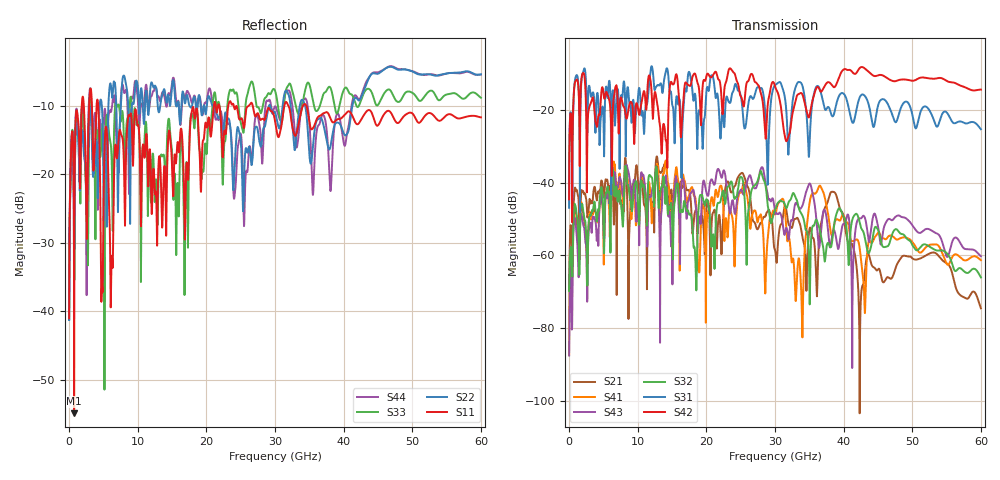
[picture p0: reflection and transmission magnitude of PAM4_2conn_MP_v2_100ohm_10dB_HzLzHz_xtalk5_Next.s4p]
! Info: Touchstone file created by Circ.  Input file=FAB50GbE_2conn_Midplane_Examax_Topo2_v2_100ohm_10dB_HzLzHz.circ
# Hz S RI R 50
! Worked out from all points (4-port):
!   6000 points, 10 MHz to 60 GHz, reference 50 ohm
!   strongest paths, dB at 10 MHz, 15.01 GHz, 30.01 GHz, 45.01 GHz, 60 GHz:
!     S42: -44.6, -12.9, -13.6, -10.6, -14.5
!     S31: -46.9, -18.4, -13.3, -19.0, -25.4
!     S32: -69.8, -50.1, -47.5, -53.0, -66.0
!     S43: -87.4, -57.1, -48.0, -52.0, -60.2
!     S41: -87.2, -45.3, -48.7, -53.7, -61.3
!     S21: -69.3, -44.4, -58.5, -63.8, -74.5
!   lowest |S11| = -54.9 dB at 740 MHz (marker M1), VSWR 1.00, Z = 49.8 + j0.0246 ohm
!   |S11| at or under -10 dB: 4.249 GHz to 21.11 GHz (16.86 GHz wide, 133 % of centre); 26.75 GHz to 31.37 GHz (4.621 GHz wide, 15.9 % of centre); 34.56 GHz to end of sweep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
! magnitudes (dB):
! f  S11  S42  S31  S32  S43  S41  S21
! 10 MHz  -41.1  -44.6  -46.9  -69.8  -87.4  -87.2  -69.3
! 740 MHz  -54.9  -14.3  -14.2  -47.3  -50.2  -47.4  -43.7
! 33.93 GHz  -10.4  -15.6  -13.1  -48.8  -46.6  -76.3  -54.2
! 36.07 GHz  -12.0  -14.0  -13.6  -50.3  -50.9  -42.6  -70.2
! 38.48 GHz  -12.5  -13.7  -21.7  -53.6  -53.4  -53.0  -42.5
! 42.39 GHz  -12.3  -8.5  -16.5  -51.3  -49.8  -58.7  -82.1
! 60 GHz  -11.7  -14.5  -25.4  -66.0  -60.2  -61.3  -74.5
